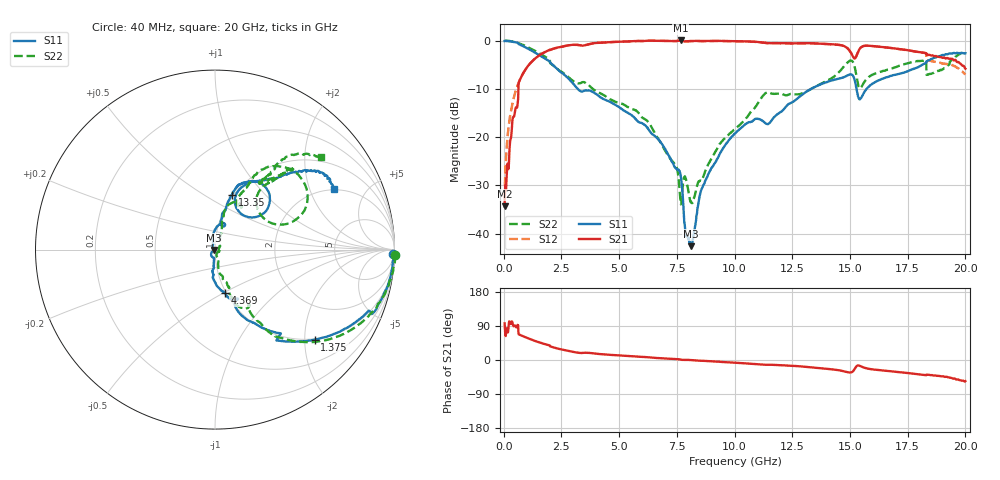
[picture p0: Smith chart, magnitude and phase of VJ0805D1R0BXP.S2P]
! VJ0805D1R0BXP
! DATE 10/29/2021  11:22
! CAPACITORS MOUNTED IN SERIES ON 25 MIL THICK MICROSTRIP SUBSTRATE
# GHz  S  MA  R  50.00
!  FREQ  S11M  S11A  S21M  S21A  S12M  S12A  S22M  S22A
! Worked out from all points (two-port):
!   1601 points, 40 MHz to 20 GHz, reference 50 ohm
!   highest |S21| = 0.06 dB at 7.662 GHz (marker M1); lowest = -34.4 dB at 40 MHz (marker M2)
!   |S21| within 3 dB of the highest: 1.57 GHz to 15.09 GHz (13.52 GHz wide, 162 % of centre); 15.3 GHz to 18.38 GHz (3.085 GHz wide, 18.3 % of centre)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
!   lowest |S11| = -42.6 dB at 8.111 GHz (marker M3), VSWR 1.01, Z = 49.3 - j0.227 ohm
!   |S11| at or under -10 dB: 3.209 GHz to 13.32 GHz (10.11 GHz wide, 122 % of centre); 15.28 GHz to 15.71 GHz (430.2 MHz wide, 2.78 % of centre)
!   |S22| runs from -34.0 to 0.1 dB; largest |S21 - S12| = 0.17
!   S11 on the Smith chart (normalised r, x): 40 MHz: 18, -79; 1.375 GHz: 0.98, -2.24; 4.369 GHz: 0.98, -0.50; 13.35 GHz: 0.98, +0.67; 20 GHz: 1.94, +2.95
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0.04  0.9946 -1.4  0.01912 96.6  0.02302 84.7  1.006 -1.6
0.21465  0.9912 -7.3  0.04804 89.3  0.1289 82.5  0.9973 -7.6
0.4392  0.9729 -15.2  0.1625 89.2  0.2566 75.3  0.9749 -15.2
0.751075  0.9009 -24.8  0.4166 65.1  0.4185 65.5  0.9233 -24.8
1.374825  0.749 -42.1  0.6594 49.8  0.658 49.8  0.7831 -40.6
3.370825  0.2974 -66.3  0.8931 18.4  0.8919 18.4  0.3678 -58.4
4.368825  0.246 -77.5  0.9621 14.8  0.9608 14.7  0.2699 -71.5
6.70165  0.0946 -93.9  0.9984 5.0  0.9975 5.0  0.09575 -78.7
7.662225  0.04052 -119.3  1.007 1.1  1.007 1.1  0.02096 -58.3
7.89925  0.009412 -125.4  0.9861 0.4  0.9829 0.2  0.03638 -34.6
8.111325  0.007393 -161.9  0.9933 -0.2  0.9917 -0.2  0.0214 -11.4
8.6228  0.03066 111.6  0.9924 -2.1  0.9915 -2.1  0.03737 47.3
10.02  0.1096 90.2  0.9911 -7.1  0.9884 -7.2  0.1215 71.6
11.3673  0.1381 69.4  0.948 -12.6  0.9475 -12.5  0.2884 66.5
13.35083  0.32 72.9  0.9426 -19.6  0.9398 -19.6  0.3201 66.1
14.82287  0.4292 62.7  0.8607 -31.1  0.8592 -31.3  0.5728 54.2
15.12228  0.437 46.7  0.691 -30.3  0.6901 -30.4  0.6056 31.9
15.44662  0.249 56.6  0.8412 -16.0  0.8392 -16.0  0.3213 39.7
16.68165  0.4248 62.0  0.8465 -29.3  0.8453 -29.4  0.5027 50.0
18.2036  0.5753 46.5  0.7502 -39.3  0.7503 -39.4  0.6219 46.3
18.61528  0.6583 41.9  0.6987 -40.9  0.6095 -36.9  0.4643 56.1
20  0.743 27.3  0.5128 -55.7  0.4465 -45.8  0.7828 41.1
